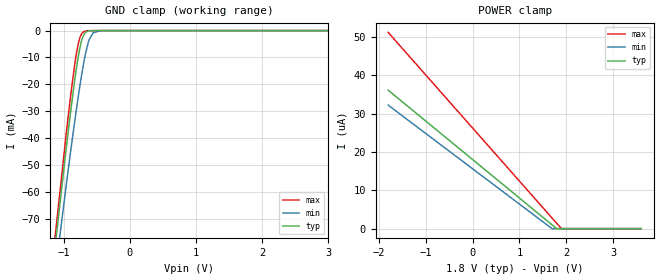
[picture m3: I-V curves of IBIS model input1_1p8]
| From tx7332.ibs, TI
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|   input1_1p8 Model
[Model]   input1_1p8
Model_type   Input
Vinl = 0.45
Vinh = 1.35
|   typ   min   max
C_comp   3.174pF   3.174pF   3.204pF
[Model spec]
|subparameter
Vinl   0.45   0.425   0.475
Vinh   1.35   1.275   1.425
| Where Nom  PVT is Nominal Process, 1.8V, 27C
|   Fast PVT is Strong Process,  1.9V, 0C
|   Slow PVT is Weak Process,   1.7V, 100C
[Voltage Range]   1.8   1.7   1.9
|Junction Temperature
[Temperature Range]   27   100   0
[Power Clamp Reference]   1.8   1.7   1.9
[GND Clamp Reference]   0   0   0
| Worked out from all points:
|   GND clamp passes 1 mA (typ) near -0.68 V on its own axis
[GND Clamp]
|   Voltage   I(typ)   I(min)   I(max)
-1.8V     -235.4mA   -228.3mA   -240.4mA
-1.136V   -82.24mA   -92.1mA    -78.7mA
-957.6mV  -43.45mA   -57.23mA   -37.99mA
-892.8mV  -30.2mA    -45.02mA   -24.31mA
-828mV    -17.96mA   -33.27mA   -12.17mA
-784.8mV  -10.83mA   -25.81mA   -5.825mA
-752.4mV  -6.417mA   -20.5mA    -2.625mA
-693mV    -1.509mA   -11.75mA   -364.4uA
-612mV    -98.47uA   -3.363mA   -28.74uA
-552.6mV  -15.9uA    -820.6uA   -10.63uA
-444.6mV  -4.627uA   -40.29uA   -6.221uA
3.6V      0A         0A         0A
[POWER Clamp]
|   Voltage   I(typ)   I(min)   I(max)
-1.8V     36.14uA    32.24uA    51.22uA
1.694V    1.043uA    32.44nA    2.833uA
1.796V    12.51nA    0A         1.412uA
1.894V    0A         0A         65.35nA
3.6V      0A         0A         0A
